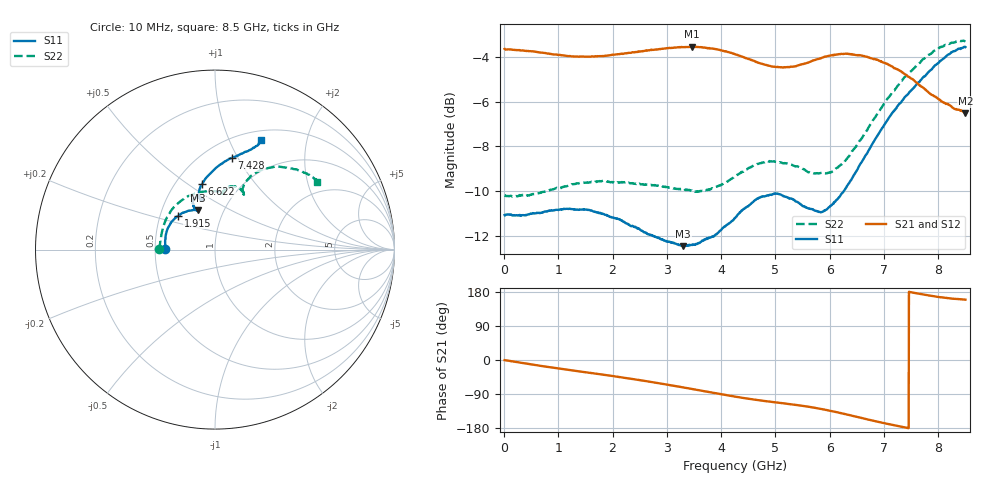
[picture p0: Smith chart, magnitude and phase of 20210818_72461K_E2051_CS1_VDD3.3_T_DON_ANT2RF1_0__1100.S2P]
!Agilent Technologies,E5071C,MY46417908,A.11.23
!Date: Wed Aug 18 14:23:11 2021
!Data & Calibration Information:
!Freq	S11:SOLT2(ON)	S21:SOLT2(ON)	S12:SOLT2(ON)	S22:SOLT2(ON)
!PortZ  Port1:50+j0  Port2:50+j0
!Above PortZ is port z conversion or system Z0 setting when saving the data.
!When reading, reference impedance value at option line is always used.
# Hz S dB R 50
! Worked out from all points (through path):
!   1601 points, 10 MHz to 8.5 GHz, reference 50 ohm
!   highest |S21| = -3.55 dB at 3.454 GHz (marker M1); lowest = -6.5 dB at 8.5 GHz (marker M2)
!   group delay of S21, straight-line fit = 66.8 ps
!   lowest |S11| = -12.5 dB at 3.3 GHz (marker M3), VSWR 1.62, Z = 37.8 + j17.5 ohm
!   |S11| at or under -10 dB: start of sweep to 6.262 GHz
!   |S22| runs from -10.3 to -3.3 dB; largest |S21 - S12| = 0.003
!   S11 on the Smith chart (normalised r, x): 10 MHz: 0.56, +0.00; 1.915 GHz: 0.62, +0.25; 6.622 GHz: 0.67, +0.57; 7.428 GHz: 0.67, +0.94; 8.5 GHz: 0.60, +1.32
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1e7  -11.08 179.7  -3.65 -0.4  -3.64 -0.4  -10.19 179.8
8.1655e8  -10.89 164.7  -3.85 -18.6  -3.85 -18.6  -9.98 153.5
1.426769e9  -10.83 150.0  -3.99 -30.9  -3.99 -30.9  -9.64 131.9
1.914944e9  -11.11 137.2  -3.94 -40.6  -3.95 -40.6  -9.59 114.7
2.334138e9  -11.57 126.7  -3.82 -49.4  -3.82 -49.5  -9.66 101.5
2.843538e9  -12.10 117.2  -3.66 -61.1  -3.66 -61.2  -9.77 89.4
3.299875e9  -12.47 113.7  -3.57 -72.3  -3.57 -72.3  -9.94 83.7
3.453756e9  -12.41 114.2  -3.55 -76.2  -3.55 -76.2  -9.98 83.2
3.862338e9  -12.04 115.9  -3.64 -86.7  -3.64 -86.7  -9.86 82.2
4.255e9  -11.22 115.8  -3.88 -96.6  -3.88 -96.6  -9.35 80.4
4.668888e9  -10.34 113.3  -4.25 -105.7  -4.24 -105.7  -8.80 75.8
4.997875e9  -10.11 109.1  -4.45 -111.7  -4.45 -111.6  -8.69 70.2
5.279106e9  -10.34 105.3  -4.44 -116.7  -4.45 -116.6  -8.81 65.1
5.671769e9  -10.82 104.3  -4.19 -124.8  -4.21 -124.8  -9.20 62.5
5.8681e9  -10.93 105.5  -4.03 -129.9  -4.05 -130.0  -9.20 63.0
6.138719e9  -10.38 107.1  -3.90 -138.0  -3.91 -138.1  -8.96 65.0
6.621588e9  -8.58 101.2  -3.96 -154.2  -3.95 -154.2  -7.53 65.5
7.088538e9  -6.73 88.6  -4.36 -169.4  -4.36 -169.5  -5.81 59.9
7.428138e9  -5.71 79.7  -4.86 -179.3  -4.86 -179.3  -4.80 53.4
8.027744e9  -4.21 68.6  -5.93 165.8  -5.89 165.9  -3.59 40.0
8.340812e9  -3.69 67.2  -6.35 160.9  -6.33 161.0  -3.30 34.9
8.5e9  -3.57 67.3  -6.54 159.2  -6.49 159.2  -3.32 33.5
